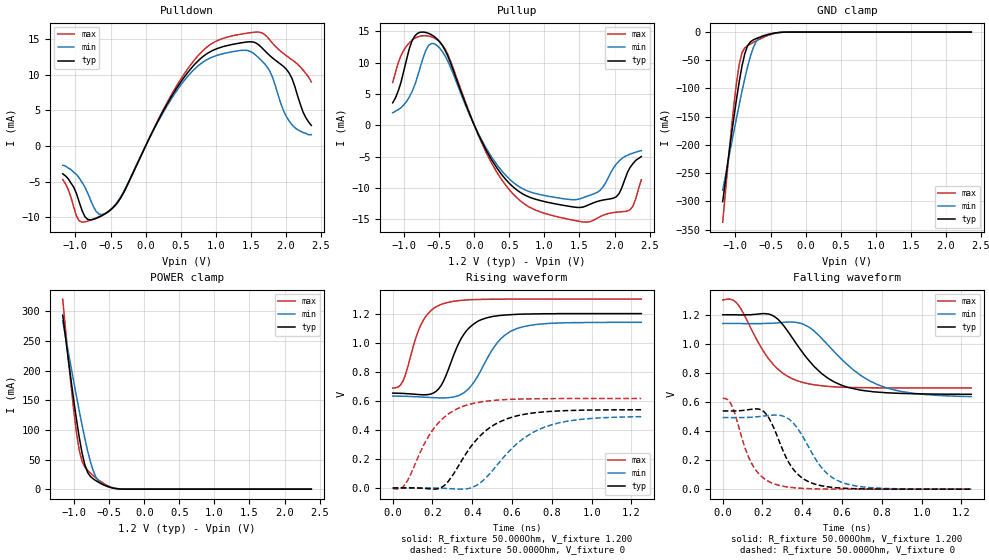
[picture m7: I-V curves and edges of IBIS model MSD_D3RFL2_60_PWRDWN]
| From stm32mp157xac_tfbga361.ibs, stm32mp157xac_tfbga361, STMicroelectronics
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[Model] MSD_D3RFL2_60_PWRDWN
Model_type   I/O
C_comp 2.581pF   2.493pF   2.708pF
Vinh = 820.000mV
Vinl = 380.000mV
Vmeas = 600.000mV
Vref = 600.000mV
[Model Spec]
Vinh   820.000mV   790.000mV   870.000mV
Vinl   380.000mV   350.000mV   430.000mV
Vmeas   600.000mV   570.000mV   650.000mV
Vref   600.000mV   570.000mV   650.000mV
[Temperature Range]   25.000   125.000   -40.000
[Voltage Range]   1.200V   1.140V   1.300V
[GND Clamp Reference]   0.00V   0.00V   0.00V
[Pulldown Reference]   0.00V   0.00V   0.00V
[POWER Clamp Reference]   1.200V   1.140V   1.300V
[Pullup Reference]   1.200V   1.140V   1.300V
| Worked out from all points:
|   slope of the pulldown table from 0 to 0.18 V, typ, clamps not added: 50.1 ohm
|   slope of the pullup table from 0 to 0.18 V, typ, clamps not added: 42.9 ohm
|   GND clamp passes 1 mA (typ) near -0.40 V on its own axis
|   POWER clamp passes 1 mA (typ) near -0.41 V on its own axis
|   rising waveform, R_fixture 50.000Ohm, V_fixture 1.200: 20-80 % time 113ps typ, 142ps min, 94.2ps max; typ from 0.653 V to 1.2 V
|   rising waveform, R_fixture 50.000Ohm, V_fixture 0: 20-80 % time 194ps typ, 232ps min, 165ps max; typ from 0 V to 0.538 V
|   falling waveform, R_fixture 50.000Ohm, V_fixture 1.200: 20-80 % time 206ps typ, 254ps min, 170ps max; typ from 1.2 V to 0.653 V
|   falling waveform, R_fixture 50.000Ohm, V_fixture 0: 20-80 % time 120ps typ, 145ps min, 104ps max; typ from 0.538 V to 0 V
[GND Clamp]
-1.182V   -300.5mA   -280.4mA   -337mA
-1.064V   -188.1mA   -202.5mA   -178.5mA
-984.9mV  -118.6mA   -152.2mA   -89.49mA
-945.5mV  -87.16mA   -127.9mA   -56.6mA
-906.1mV  -59.71mA   -104.4mA   -36.4mA
-866.7mV  -38.14mA   -82.14mA   -27.92mA
-827.3mV  -24.29mA   -61.54mA   -24.05mA
-748.5mV  -14mA      -28.45mA   -18.47mA
-709.1mV  -11.76mA   -17.8mA    -15.89mA
-630.3mV  -8.132mA   -7.75mA    -11.05mA
-472.7mV  -2.557mA   -2.242mA   -3.323mA
2.364V    29.58nA    484.6nA    2.864nA
[Power Clamp]
-1.164V   293.6mA    283.6mA    320.6mA
-1.085V   219.6mA    231.9mA    221.3mA
-1.006V   149.3mA    180.9mA    132.2mA
-966.7mV  116.7mA    156mA      94.33mA
-927.3mV  86.87mA    131.6mA    64.9mA
-887.9mV  61.07mA    108mA      46.71mA
-809.1mV  28.38mA    64.84mA    31.83mA
-730.3mV  17.49mA    31.58mA    22.97mA
-651.5mV  11.58mA    13.7mA     15.38mA
-533.3mV  4.956mA    4.897mA    6.46mA
-336.4mV  215.7uA    403.7uA    242.8uA
2.382V    -24.83nA   -515.5nA   -2.721nA
[Pulldown]
-1.182V   -3.9mA     -2.7mA     -4.7mA
-945.5mV  -7.91mA    -4.5mA     -10.51mA
-827.3mV  -10.3mA    -6.57mA    -10.56mA
-669.7mV  -10.02mA   -9.53mA    -9.95mA
-551.5mV  -9.376mA   -9.339mA   -9.297mA
-315.1mV  -6.567mA   -6.464mA   -6.607mA
551.5mV   9.679mA    9.198mA    10.14mA
906.1mV   13.16mA    12.3mA     14.14mA
1.261V    14.32mA    13.29mA    15.53mA
1.733V    13.06mA    11.13mA    15.34mA
2.009V    10.78mA    4.13mA     12.68mA
2.364V    2.9mA      1.6mA      9mA
[Pullup]
-1.164V   3.6mA      2.005mA    6.838mA
-1.045V   6.9mA      2.809mA    11.16mA
-887.9mV  13.52mA    5.386mA    13.61mA
-690.9mV  14.84mA    11.99mA    14.32mA
-454.5mV  12.73mA    11.77mA    12.85mA
175.8mV   -4.107mA   -3.772mA   -4.491mA
687.9mV   -10.95mA   -10.13mA   -12.35mA
1.476V    -13.13mA   -11.84mA   -15.31mA
1.791V    -12.06mA   -10.42mA   -14.62mA
1.988V    -11.63mA   -6.784mA   -13.95mA
2.224V    -6.7mA     -4.595mA   -13.48mA
2.382V    -5mA       -4.048mA   -8.7mA
[Ramp]
R_load=50.000Ohm
dV/dt_r   325.740mV/154.000ps  300.149mV/188.500ps  366.060mV/130.000ps
dV/dt_f   325.740mV/164.000ps  300.089mV/203.000ps  366.060mV/137.000ps
[Rising waveform]
R_fixture=50.000Ohm
V_fixture=1.200
V_fixture_min=1.140
V_fixture_max=1.300
0s        652.7mV    632.7mV    687.5mV
52ps      650.6mV    631.3mV    736.8mV
115ps     644.6mV    627.9mV    1.028V
154ps     641.2mV    625.2mV    1.154V
243ps     703.8mV    619.7mV    1.263V
345ps     1.03V      645.3mV    1.291V
447ps     1.159V     818mV      1.298V
537ps     1.187V     1.017V     1.299V
626ps     1.195V     1.098V     1.3V
1.25ns    1.2V       1.14V      1.3V
[Rising waveform]
R_fixture=50.000Ohm
V_fixture=0
0s        162.9uV    126.8uV    -3.342mV
64ps      665.4uV    472.6uV    27.93mV
166ps     -3.839mV   609.5uV    321.3mV
243ps     1.833mV    -1.609mV   467.1mV
358ps     213.5mV    -7.703mV   563.7mV
422ps     333.1mV    18.16mV    586.3mV
511ps     435.5mV    134.7mV    603mV
626ps     497.2mV    306.3mV    611.3mV
754ps     523.1mV    413.3mV    614.4mV
1.25ns    538.2mV    490.7mV    616mV
[Falling waveform]
R_fixture=50.000Ohm
V_fixture=1.200
V_fixture_min=1.140
V_fixture_max=1.300
0s        1.2V       1.14V      1.302V
77ps      1.199V     1.14V      1.27V
243ps     1.2V       1.141V     876.9mV
294ps     1.145V     1.146V     806.5mV
371ps     998.9mV    1.147V     748.1mV
498ps     795mV      1.037V     711.5mV
626ps     701.9mV    858mV      700.4mV
741ps     672.9mV    743.5mV    697.6mV
843ps     662.1mV    689.7mV    696.7mV
1.25ns    653mV      637mV      696.2mV
[Falling waveform]
R_fixture=50.000Ohm
V_fixture=0
0s        538.1mV    492.8mV    625.1mV
52ps      537.9mV    492.4mV    554.8mV
154ps     551.4mV    496mV      156.3mV
205ps     535.9mV    502.9mV    76.01mV
256ps     424.3mV    509.6mV    37.97mV
345ps     155.6mV    468.4mV    11.7mV
460ps     36.05mV    221.8mV    2.626mV
549ps     12.78mV    81.56mV    830.5uV
664ps     3.345mV    23.25mV    248.4uV
1.25ns    21.39uV    54.29uV    -7.986uV
